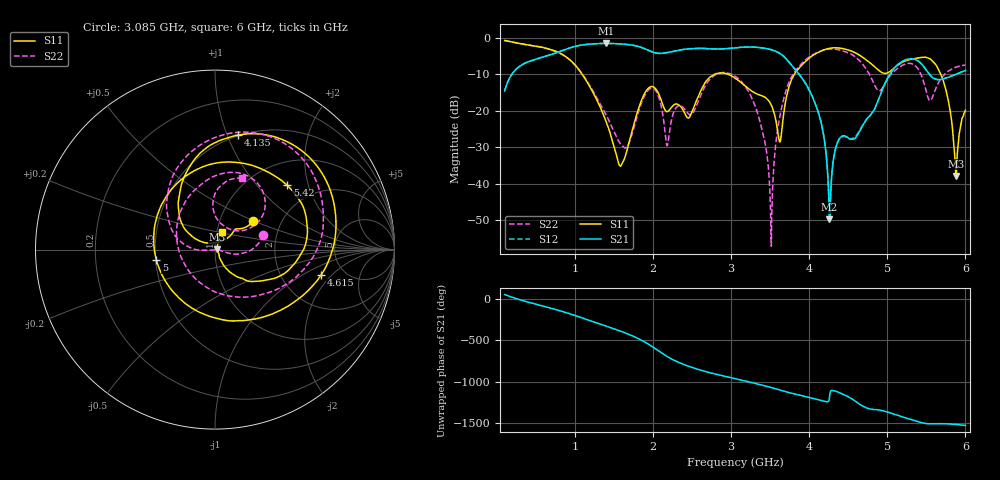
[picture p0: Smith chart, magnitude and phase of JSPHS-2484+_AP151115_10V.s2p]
!Mini-Circuits Laboratory
!S-Parameters
!Run/Lot/Date Code:MF33450/NA/1551
!Fixture/SN/Due: 90-4-20-21/70546/03/17/16
!Connection:PORT<IN> - pin<1>; PORT<OUT> - pin<7>;PORT<BIAS> - pin<4>;
!Tested With:PORT EXTENTION
!Network Analyzer:AG E5071C/74883/05/12/16
!Created: 01-07-2016 at 14:10:37
!MODEL: JSPHS-2484+
!S/N: V=10V
# MHZ S DB R 50
!Frequency  S11 dB  S11 DEG  S21 dB  S21 DEG  S12 dB  S12 DEG  S22 dB  S22 DEG
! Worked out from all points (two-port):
!   1181 points, 100 MHz to 6 GHz, reference 50 ohm
!   highest |S21| = -1.48 dB at 1.395 GHz (marker M1); lowest = -49.8 dB at 4.26 GHz (marker M2)
!   |S21| within 3 dB of the highest: 704.3 MHz to 3.642 GHz (2.937 GHz wide, 135 % of centre)
!   lowest |S11| = -37.9 dB at 5.88 GHz (marker M3), VSWR 1.03, Z = 51.3 + j0.243 ohm
!   |S11| at or under -10 dB: 1.095 GHz to 2.784 GHz (1.689 GHz wide, 87.1 % of centre); 2.965 GHz to 3.809 GHz (844.1 MHz wide, 24.9 % of centre); 5.685 GHz to end of sweep
!   |S22| runs from -57.1 to -0.7 dB; largest |S21 - S12| = 0.0054
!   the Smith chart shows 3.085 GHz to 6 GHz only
!   S11 on the Smith chart (normalised r, x): 3.085 GHz: 1.43, +0.50; 4.135 GHz: 0.49, +1.09; 4.615 GHz: 3.36, -1.51; 5 GHz: 0.50, -0.07; 5.42 GHz: 1.46, +1.48; 6 GHz: 1.06, +0.20
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100  -0.67 -37.5  -14.56 52.2  -14.55 52.1  -0.66 -37.5
540  -2.37 -162.4  -5.54 -74.3  -5.54 -74.4  -2.41 -165.8
1085  -9.68 48.3  -1.93 132.3  -1.93 132.3  -9.65 43.2
1395  -22.71 -50.4  -1.48 32.5  -1.47 32.5  -20.92 -72.3
1740  -24.99 139.6  -1.97 -88.6  -1.96 -88.6  -25.81 173.2
1915  -14.44 83.4  -3.13 -172.6  -3.12 -172.7  -14.99 96.6
2070  -15.19 24.5  -4.21 92.2  -4.21 92.1  -15.98 15.1
2235  -19.10 45.7  -3.76 -5.0  -3.76 -5.1  -22.73 76.2
2450  -21.95 60.4  -2.97 -92.6  -2.97 -92.7  -20.76 55.7
3050  -11.00 39.5  -2.70 116.9  -2.70 116.8  -10.46 22.4
3085  -11.52 37.6  -2.62 109.2  -2.63 109.2  -11.04 16.6
3515  -18.43 42.6  -3.21 8.4  -3.22 8.3  -57.15 -122.7
3685  -19.04 151.0  -5.26 -37.7  -5.27 -37.8  -15.74 171.8
4035  -4.94 95.2  -15.77 -120.0  -15.85 -119.2  -4.74 99.9
4135  -3.73 78.6  -21.76 -144.1  -21.73 -143.4  -3.66 82.0
4260  -2.82 56.5  -49.79 -110.3  -49.55 -111.4  -3.03 59.0
4615  -4.33 -13.5  -26.65 -172.3  -26.32 -172.4  -5.64 -9.2
5000  -9.59 -170.0  -11.18 73.1  -11.19 72.9  -11.38 139.1
5020  -9.37 177.8  -10.39 67.2  -10.40 67.0  -10.74 130.5
5420  -5.37 41.7  -6.73 -51.2  -6.73 -51.2  -9.46 36.6
5880  -37.85 10.7  -9.95 -77.6  -9.95 -77.8  -7.97 77.7
6000  -19.83 69.2  -8.88 -89.6  -8.87 -89.5  -7.44 68.9
